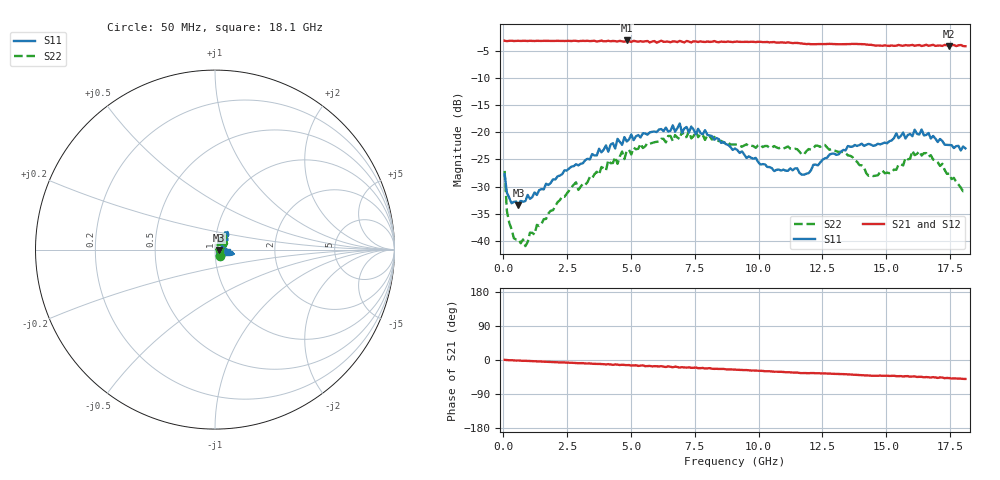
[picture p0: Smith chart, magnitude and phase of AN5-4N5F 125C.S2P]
! Network Analyzer HP8720D.06.14 Serial No. US36140669
! 28 Jun 2005  13:06:36
! Frequency  S11  S21  S12  S22
# HZ  S  DB R 50
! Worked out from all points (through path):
!   201 points, 50 MHz to 18.1 GHz, reference 50 ohm
!   highest |S21| = -3.10 dB at 4.833 GHz (marker M1); lowest = -4.2 dB at 17.47 GHz (marker M2)
!   group delay of S21, straight-line fit = 7.73 ps
!   lowest |S11| = -33.5 dB at 591.5 MHz (marker M3), VSWR 1.04, Z = 52.2 - j0.215 ohm
!   |S11| at or under -10 dB: start of sweep to end of sweep
!   |S22| runs from -41.0 to -19.7 dB; largest |S21 - S12| = 0.023
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5e7  -27.75 -50.3  -3.15 0.4  -3.16 0.4  -27.11 -54.6
1.4025e8  -31.13 -34.1  -3.23 -0.1  -3.21 -0.2  -34.49 -52.4
2.305e8  -32.03 -22.4  -3.17 -0.6  -3.16 -0.6  -36.64 -45.0
5.915e8  -33.46 -5.6  -3.16 -1.3  -3.20 -1.4  -39.69 -3.4
8.6225e8  -32.65 0.6  -3.17 -2.1  -3.20 -2.3  -40.96 14.8
2.30625e9  -27.70 18.1  -3.19 -6.4  -3.19 -6.4  -31.77 51.0
3.1185e9  -25.68 29.4  -3.17 -8.3  -3.21 -8.6  -29.45 60.9
4.83325e9  -21.70 47.6  -3.10 -13.5  -3.22 -13.8  -23.37 57.7
6.09675e9  -19.49 49.0  -3.32 -17.1  -3.23 -17.1  -21.70 59.7
6.909e9  -18.38 54.6  -3.18 -20.0  -3.22 -18.9  -21.25 56.1
7.27e9  -20.06 54.6  -3.30 -19.4  -3.39 -20.8  -19.73 56.7
9.075e9  -22.99 54.4  -3.33 -25.5  -3.31 -25.6  -22.25 40.4
1.060925e10  -27.14 33.0  -3.38 -30.9  -3.45 -31.1  -22.53 27.0
1.17825e10  -27.79 7.1  -3.71 -34.4  -3.70 -34.8  -24.03 43.3
1.21435e10  -25.98 12.7  -3.79 -34.5  -3.74 -34.8  -22.92 48.8
1.3407e10  -23.33 -5.8  -3.76 -37.5  -3.74 -37.7  -23.78 47.4
1.43095e10  -22.13 -22.0  -3.90 -41.0  -3.86 -41.3  -28.01 43.0
1.512175e10  -21.64 -14.1  -4.11 -42.1  -3.99 -42.1  -27.52 45.9
1.602425e10  -20.72 -13.1  -3.91 -43.5  -4.08 -44.8  -23.39 28.8
1.638525e10  -19.48 -13.3  -4.12 -44.5  -3.91 -44.7  -24.28 19.4
1.746825e10  -22.34 -11.4  -4.16 -47.7  -4.16 -47.9  -27.62 1.8
1.81e10  -22.95 -12.3  -4.16 -50.0  -4.18 -50.5  -30.67 -20.1
